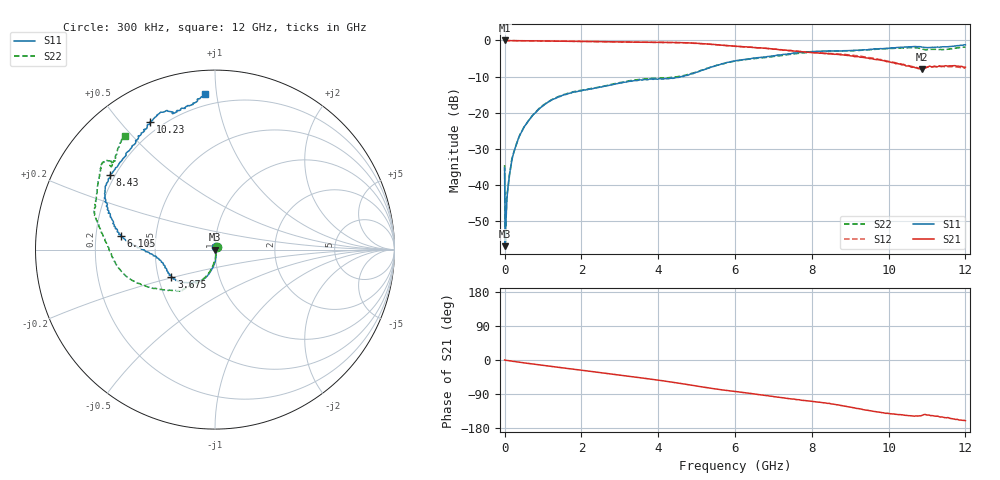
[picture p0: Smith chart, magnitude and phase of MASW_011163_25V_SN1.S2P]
!Agilent Technologies,E5071C,MY46418240,A.11.23
!Date: Mon Dec 07 11:49:18 2020
!Data & Calibration Information:
!Freq	S11:SOLT2(ON)	S21:SOLT2(ON)	S12:SOLT2(ON)	S22:SOLT2(ON)
!PortZ  Port1:50+j0  Port2:50+j0
!Above PortZ is port z conversion or system Z0 setting when saving the data.
!When reading, reference impedance value at option line is always used.
# Hz S dB R 50
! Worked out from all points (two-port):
!   801 points, 300 kHz to 12 GHz, reference 50 ohm
!   highest |S21| = -0.02 dB at 300 kHz (marker M1); lowest = -8.0 dB at 10.88 GHz (marker M2)
!   |S21| within 3 dB of the highest: start of sweep to 7.631 GHz
!   lowest |S11| = -57.0 dB at 15.3 MHz (marker M3), VSWR 1.00, Z = 50.1 - j0.0236 ohm
!   |S11| at or under -10 dB: start of sweep to 4.632 GHz
!   |S22| runs from -56.5 to -1.8 dB; largest |S21 - S12| = 0.043
!   S11 on the Smith chart (normalised r, x): 300 kHz: 1.01, +0.03; 3.675 GHz: 0.59, -0.20; 6.105 GHz: 0.31, +0.07; 8.43 GHz: 0.18, +0.31; 10.23 GHz: 0.15, +0.60; 12 GHz: 0.13, +0.93
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300000  -35.34 66.9  -0.02 0.1  -0.02 0.2  -34.54 60.7
1.529962e7  -56.96 -9.5  -0.06 -0.4  -0.06 -0.3  -56.46 -56.8
7.529812e7  -42.01 -54.0  -0.06 -1.4  -0.06 -1.4  -41.87 -58.6
1.052974e8  -39.03 -59.9  -0.06 -1.8  -0.06 -1.8  -39.03 -62.3
1.502962e8  -35.50 -65.6  -0.07 -2.5  -0.07 -2.5  -36.02 -65.5
2.852929e8  -29.47 -79.8  -0.08 -4.5  -0.07 -4.5  -29.46 -83.0
4.352891e8  -25.46 -86.6  -0.09 -6.6  -0.09 -6.6  -25.37 -88.5
6.452839e8  -21.95 -92.6  -0.11 -9.5  -0.11 -9.5  -21.90 -95.8
1.20027e9  -16.69 -105.4  -0.19 -16.8  -0.19 -16.8  -16.58 -107.1
2.01025e9  -13.93 -118.4  -0.29 -27.1  -0.29 -27.1  -13.78 -116.8
3.675208e9  -10.84 -147.6  -0.52 -48.7  -0.53 -48.8  -10.63 -129.3
4.0052e9  -10.72 -155.6  -0.55 -53.2  -0.56 -53.3  -10.48 -130.0
4.995175e9  -8.82 -176.3  -0.80 -68.6  -0.82 -68.8  -8.71 -142.2
6.00015e9  -5.68 172.3  -1.60 -83.0  -1.63 -83.5  -5.72 -163.4
6.105147e9  -5.50 171.6  -1.68 -84.3  -1.70 -84.9  -5.56 -165.3
8.0101e9  -3.08 150.7  -3.38 -109.1  -3.34 -110.3  -3.23 165.0
8.430089e9  -2.89 144.4  -3.76 -114.3  -3.59 -115.8  -3.01 162.2
1.000505e10  -2.20 119.3  -5.91 -141.1  -5.82 -139.8  -2.27 146.5
1.023004e10  -1.96 116.8  -6.43 -143.9  -6.33 -142.0  -2.14 144.7
1.087503e10  -1.86 107.9  -7.95 -145.7  -7.87 -141.8  -2.39 139.6
1.146001e10  -1.76 100.6  -7.08 -152.1  -7.27 -146.9  -2.52 137.8
1.2e10  -1.21 93.8  -7.40 -160.2  -7.74 -155.7  -1.84 128.2
